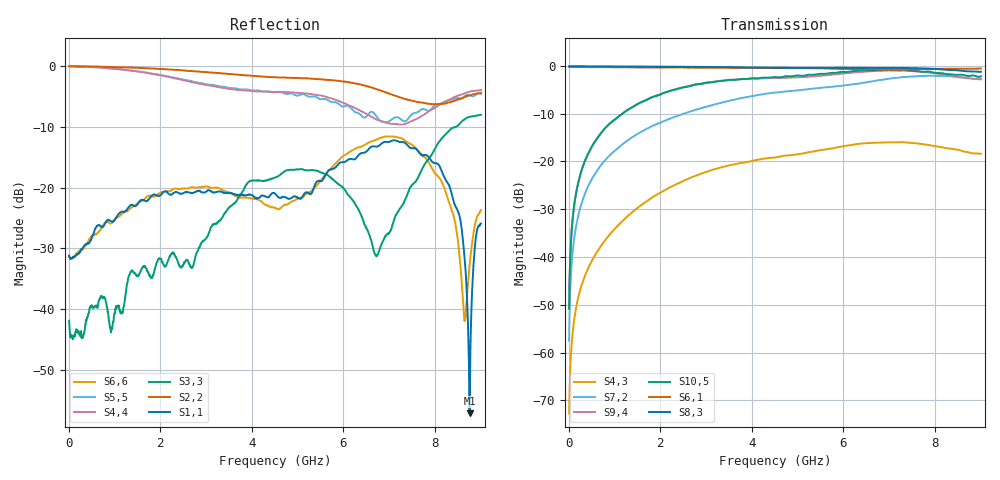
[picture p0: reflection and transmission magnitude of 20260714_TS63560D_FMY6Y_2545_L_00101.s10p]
# GHz S DB R 50
! CMT, SN0916, 25263762, 26.7.0
! Date: 15.07.2026 13:34:48
! Data: Format
! Freq S1.1:dB/Ang S1.2:dB/Ang S1.3:dB/Ang S1.4:dB/Ang S1.5:dB/Ang S1.6:dB/Ang S1.7:dB/Ang S1.8:dB/Ang S1.9:dB/Ang S1.10:dB/Ang
!  S2.1:dB/Ang S2.2:dB/Ang S2.3:dB/Ang S2.4:dB/Ang S2.5:dB/Ang S2.6:dB/Ang S2.7:dB/Ang S2.8:dB/Ang S2.9:dB/Ang S2.10:dB/Ang
!  S3.1:dB/Ang S3.2:dB/Ang S3.3:dB/Ang S3.4:dB/Ang S3.5:dB/Ang S3.6:dB/Ang S3.7:dB/Ang S3.8:dB/Ang S3.9:dB/Ang S3.10:dB/Ang
!  S4.1:dB/Ang S4.2:dB/Ang S4.3:dB/Ang S4.4:dB/Ang S4.5:dB/Ang S4.6:dB/Ang S4.7:dB/Ang S4.8:dB/Ang S4.9:dB/Ang S4.10:dB/Ang
!  S5.1:dB/Ang S5.2:dB/Ang S5.3:dB/Ang S5.4:dB/Ang S5.5:dB/Ang S5.6:dB/Ang S5.7:dB/Ang S5.8:dB/Ang S5.9:dB/Ang S5.10:dB/Ang
!  S6.1:dB/Ang S6.2:dB/Ang S6.3:dB/Ang S6.4:dB/Ang S6.5:dB/Ang S6.6:dB/Ang S6.7:dB/Ang S6.8:dB/Ang S6.9:dB/Ang S6.10:dB/Ang
!  S7.1:dB/Ang S7.2:dB/Ang S7.3:dB/Ang S7.4:dB/Ang S7.5:dB/Ang S7.6:dB/Ang S7.7:dB/Ang S7.8:dB/Ang S7.9:dB/Ang S7.10:dB/Ang
!  S8.1:dB/Ang S8.2:dB/Ang S8.3:dB/Ang S8.4:dB/Ang S8.5:dB/Ang S8.6:dB/Ang S8.7:dB/Ang S8.8:dB/Ang S8.9:dB/Ang S8.10:dB/Ang
!  S9.1:dB/Ang S9.2:dB/Ang S9.3:dB/Ang S9.4:dB/Ang S9.5:dB/Ang S9.6:dB/Ang S9.7:dB/Ang S9.8:dB/Ang S9.9:dB/Ang S9.10:dB/Ang
!  S10.1:dB/Ang S10.2:dB/Ang S10.3:dB/Ang S10.4:dB/Ang S10.5:dB/Ang S10.6:dB/Ang S10.7:dB/Ang S10.8:dB/Ang S10.9:dB/Ang S10.10:dB/Ang
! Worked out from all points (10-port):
!   2001 points, 10 MHz to 9 GHz, reference 50 ohm
!   strongest paths, dB at 10 MHz, 2.257 GHz, 4.505 GHz, 6.753 GHz, 9 GHz:
!     S8,3: -0.1, -0.2, -0.4, -0.4, -1.3
!     S6,1: -0.2, -0.4, -0.5, -0.8, -0.6
!     S10,5: -50.8, -5.1, -2.3, -0.8, -2.2
!     S9,4: -50.9, -5.1, -2.6, -1.0, -2.8
!     S7,2: -57.5, -10.9, -5.6, -3.0, -2.7
!     S4,3: -72.7, -25.2, -19.2, -16.1, -18.4
!   lowest |S11| = -57.2 dB at 8.753 GHz (marker M1), VSWR 1.00, Z = 50 - j0.138 ohm
!   |S11| at or under -10 dB: start of sweep to end of sweep
